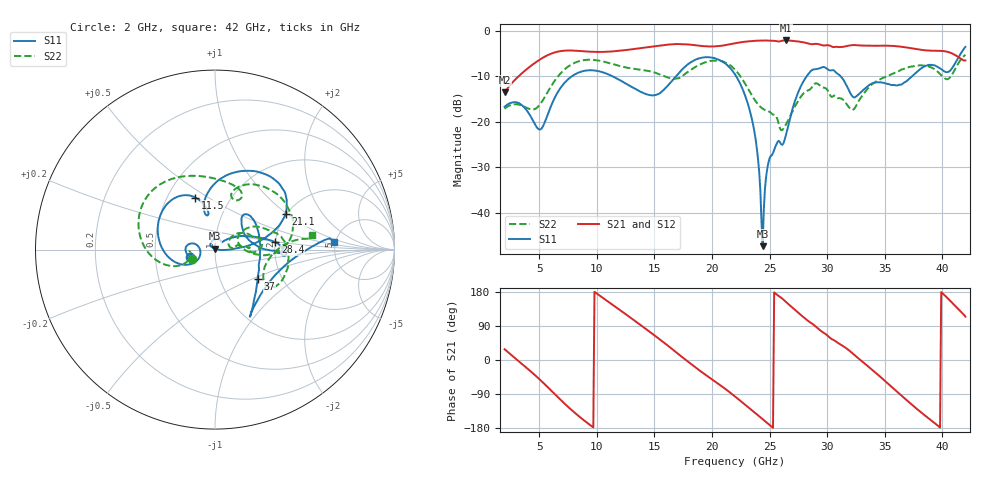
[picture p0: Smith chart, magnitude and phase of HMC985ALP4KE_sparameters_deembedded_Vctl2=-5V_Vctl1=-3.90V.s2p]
!s2p File: Measurements: S11, S21, S12, S22
# GHz S dB R 50.0
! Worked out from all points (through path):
!   401 points, 2 GHz to 42 GHz, reference 50 ohm
!   highest |S21| = -2.13 dB at 26.4 GHz (marker M1); lowest = -13.5 dB at 2 GHz (marker M2)
!   lowest |S11| = -47.3 dB at 24.4 GHz (marker M3), VSWR 1.01, Z = 49.9 + j0.427 ohm
!   |S11| at or under -10 dB: start of sweep to 7.844 GHz; 22.1 GHz to 28.22 GHz (6.123 GHz wide, 24.3 % of centre); 31.17 GHz to 37.37 GHz (6.199 GHz wide, 18.1 % of centre)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
!   |S22| runs from -21.9 to -5.3 dB; largest |S21 - S12| = 0.00097
!   S11 on the Smith chart (normalised r, x): 2 GHz: 0.75, -0.06; 11.5 GHz: 0.69, +0.44; 21.1 GHz: 1.97, +0.98; 28.4 GHz: 2.00, +0.19; 37 GHz: 1.51, -0.53; 42 GHz: 4.86, +0.74
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2  -16.70 -163.2  -13.52 28.4  -13.53 28.4  -17.15 -158.0
5.1  -21.68 -170.3  -6.27 -52.9  -6.27 -52.9  -16.10 -158.9
6.3  -14.98 -151.7  -4.81 -88.3  -4.81 -88.3  -11.16 -161.4
8.7  -8.94 149.8  -4.48 -154.7  -4.48 -154.7  -6.54 151.4
11.5  -10.17 110.7  -4.51 142.9  -4.51 142.9  -7.40 105.4
13.6  -13.13 100.6  -3.89 96.8  -3.90 96.8  -8.50 76.4
15.4  -13.83 105.1  -3.30 56.0  -3.30 56.0  -9.52 63.2
17.9  -7.38 79.5  -3.01 -4.0  -3.01 -4.0  -9.05 71.9
21.1  -7.10 27.1  -3.19 -74.9  -3.18 -74.9  -6.91 15.8
22  -9.57 16.6  -2.75 -96.2  -2.75 -96.2  -8.54 0.6
23.5  -19.77 2.2  -2.26 -133.5  -2.26 -133.5  -14.33 -4.4
24.4  -47.31 97.2  -2.15 -156.2  -2.15 -156.1  -17.11 7.7
25  -28.02 130.9  -2.18 -171.4  -2.18 -171.4  -17.80 10.7
26.4  -23.13 44.2  -2.13 153.8  -2.13 153.9  -20.68 32.6
28.4  -9.40 7.1  -2.83 101.8  -2.83 101.9  -13.04 18.2
28.7  -8.60 1.9  -2.96 95.7  -2.96 95.7  -12.28 16.5
30.7  -8.98 -3.2  -3.54 50.3  -3.54 50.3  -14.31 2.7
32.4  -14.64 30.0  -3.15 12.4  -3.15 12.4  -16.96 26.7
35.4  -11.77 18.0  -3.30 -65.5  -3.29 -65.5  -9.78 19.0
37  -10.84 -34.2  -3.72 -108.6  -3.72 -108.5  -8.06 4.7
39.8  -8.25 -56.2  -4.42 -178.3  -4.42 -178.2  -9.48 -34.0
42  -3.54 3.6  -6.53 114.3  -6.53 114.4  -5.26 8.4
